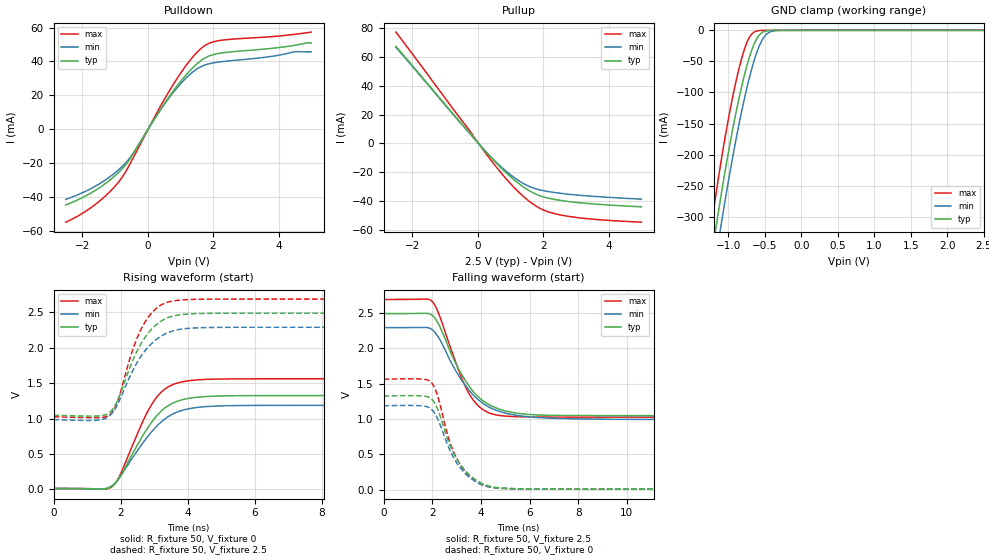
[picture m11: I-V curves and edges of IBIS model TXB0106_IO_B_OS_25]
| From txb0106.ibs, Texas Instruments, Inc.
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[Model]   TXB0106_IO_B_OS_25
Model_type  I/O
Vinl=0.804
Vinh=1.755
Enable   Active-High
Vref =   0
Rref =   1e6
Cref =   15p
Vmeas =   1.25
| variable   typ   min   max
C_comp   14.10pF   12.01pF   15.65pF
| C_pullup   14.56pF   11.56pF   16.88pF
| C_pulldown   14.64pF   13.21pF   15.28pF
| C_tri-state   14.10pF   12.01pF   15.65pF
[Temperature Range]   40   100   -40
| Ambient temperature   25   85   -40
[Voltage range]   2.5   2.3   2.7
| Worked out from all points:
|   slope of the pulldown table from 0 to 0.375 V, typ, clamps not added: 32.3 ohm
|   slope of the pullup table from 0 to 0.375 V, typ, clamps not added: 38.8 ohm
|   GND clamp passes 1 mA (typ) near -0.48 V on its own axis
|   rising waveform, R_fixture 50, V_fixture 0: 20-80 % time 1.03ns typ, 1.13ns min, 905ps max; typ from 0.011 V to 1.32 V
|   falling waveform, R_fixture 50, V_fixture 2.5: 20-80 % time 1.38ns typ, 1.53ns min, 1.11ns max; typ from 2.49 V to 1.05 V
|   rising waveform, R_fixture 50, V_fixture 2.5: 20-80 % time 830ps typ, 904ps min, 730ps max; typ from 1.05 V to 2.49 V
|   falling waveform, R_fixture 50, V_fixture 0: 20-80 % time 1.04ns typ, 1.03ns min, 938ps max; typ from 1.32 V to 0.011 V
[GND Clamp]
| TXB0104_IO_B_OS_25
|   Voltage   I(typ)   I(min)   I(max)
-2.5V     -1.624A    -1.631A    -1.656A
-1.23V    -364.1mA   -412.3mA   -311.6mA
-1.165V   -313.6mA   -361.9mA   -259.8mA
-1.095V   -262mA     -309.8mA   -207.4mA
-955mV    -168.1mA   -213.3mA   -115.3mA
-840mV    -101.9mA   -142.9mA   -55.01mA
-735mV    -52.54mA   -87.17mA   -16.66mA
-640mV    -20.26mA   -46.01mA   -2.365mA
-580mV    -8.156mA   -26.2mA    -431.3uA
-520mV    -2.458mA   -12.36mA   -59.71uA
-375mV    -59.94uA   -836.3uA   -194.6nA
2.5V      653.8pA    127nA      69.91pA
[Pulldown]
| TXB0104_IO_B_OS_25
|   Voltage   I(typ)   I(min)   I(max)
-2.5V     -44.85mA   -41.54mA   -55.03mA
-1.59V    -36.15mA   -33.67mA   -44.42mA
-860mV    -25.14mA   -23.58mA   -30.62mA
-490mV    -16.17mA   -15.63mA   -18.81mA
290mV     8.469mA    8.333mA    9.879mA
775mV     22.26mA    21.42mA    26.05mA
1.265V    33.93mA    31.83mA    39.87mA
1.68V     41.12mA    37.33mA    48.38mA
2.24V     44.92mA    39.77mA    52.45mA
3.745V    47.62mA    42.84mA    54.55mA
4.51V     49.53mA    45.76mA    56.04mA
5V        50.89mA    45.65mA    57.32mA
[Pullup]
| TXB0104_IO_B_OS_25
|   Voltage   I(typ)   I(min)   I(max)
-2.5V     67.26mA    66.61mA    77.22mA
-655mV    17.92mA    17.51mA    20.97mA
345mV     -8.329mA   -8.075mA   -9.952mA
685mV     -16.41mA   -15.67mA   -19.69mA
1.005V    -23.23mA   -21.86mA   -28.03mA
1.3V      -28.68mA   -26.58mA   -34.83mA
1.58V     -32.92mA   -29.95mA   -40.31mA
1.81V     -35.56mA   -31.79mA   -43.91mA
2.03V     -37.32mA   -32.94mA   -46.46mA
2.59V     -39.8mA    -34.83mA   -49.95mA
3.49V     -41.98mA   -36.69mA   -52.58mA
5V        -44.05mA   -38.73mA   -54.71mA
[Ramp]
| TXB0104_IO_B_OS_25
| variable   typ   min   max
dV/dt_r   0.79/1.03E-09   0.71/1.13E-09   0.94/9.11E-10
dV/dt_f   0.87/1.38E-09   0.78/1.53E-09   1.00/1.11E-09
R_load = 50
[Rising Waveform]
| TXB0104_IO_B_OS_25
R_fixture =   50
C_fixture =   0
L_fixture =   0
V_fixture =   0
V_fixture_min = 0
V_fixture_max = 0
|   Time   V(typ)   V(min)   V(max)
0s        11.18mV    9.66mV     11.79mV
1.42ns    3.203mV    3.755mV    3.327mV
1.735ns   40.8mV     48.58mV    34.72mV
1.96ns    161.8mV    160.1mV    178.6mV
2.7ns     787mV      677.5mV    997.2mV
3.075ns   1.037V     890.9mV    1.3V
3.53ns    1.211V     1.057V     1.473V
4.24ns    1.298V     1.154V     1.544V
6.495ns   1.324V     1.186V     1.561V
39.89ns   1.325V     1.186V     1.561V
[Falling Waveform]
| TXB0104_IO_B_OS_25
R_fixture =   50
C_fixture =   0
L_fixture =   0
V_fixture =   2.5
V_fixture_min = 2.3
V_fixture_max = 2.7
|   Time   V(typ)   V(min)   V(max)
0s        2.487V     2.289V     2.687V
1.995ns   2.462V     2.26V      2.658V
2.25ns    2.343V     2.154V     2.5V
3.13ns    1.677V     1.587V     1.645V
3.54ns    1.45V      1.395V     1.341V
4.1ns     1.254V     1.216V     1.128V
4.825ns   1.131V     1.1V       1.047V
6.09ns    1.061V     1.027V     1.028V
8.74ns    1.048V     998mV      1.026V
39.89ns   1.047V     987.1mV    1.025V
[Rising Waveform]
| TXB0104_IO_B_OS_25
R_fixture =   50
C_fixture =   0
L_fixture =   0
V_fixture =   2.5
V_fixture_min = 2.3
V_fixture_max = 2.7
|   Time   V(typ)   V(min)   V(max)
0s        1.047V     985.3mV    1.025V
1.32ns    1.036V     977.6mV    1.013V
1.7ns     1.098V     1.052V     1.065V
1.905ns   1.249V     1.197V     1.235V
2.37ns    1.826V     1.683V     1.982V
2.725ns   2.144V     1.955V     2.359V
3.175ns   2.365V     2.153V     2.594V
3.77ns    2.465V     2.26V      2.672V
5.685ns   2.487V     2.288V     2.687V
39.89ns   2.487V     2.289V     2.687V
[Falling Waveform]
| TXB0104_IO_B_OS_25
R_fixture =   50
C_fixture =   0
L_fixture =   0
V_fixture =   0
V_fixture_min = 0
V_fixture_max = 0
|   Time   V(typ)   V(min)   V(max)
0s        1.325V     1.186V     1.561V
1.515ns   1.326V     1.186V     1.564V
1.93ns    1.291V     1.147V     1.525V
2.075ns   1.236V     1.093V     1.453V
2.21ns    1.146V     1.01V      1.334V
2.74ns    618mV      546.5mV    657.3mV
3.115ns   376.8mV    326.5mV    377.5mV
3.77ns    144.7mV    118.8mV    123.4mV
4.55ns    37.69mV    30.88mV    30.51mV
39.89ns   11.18mV    9.66mV     11.79mV
